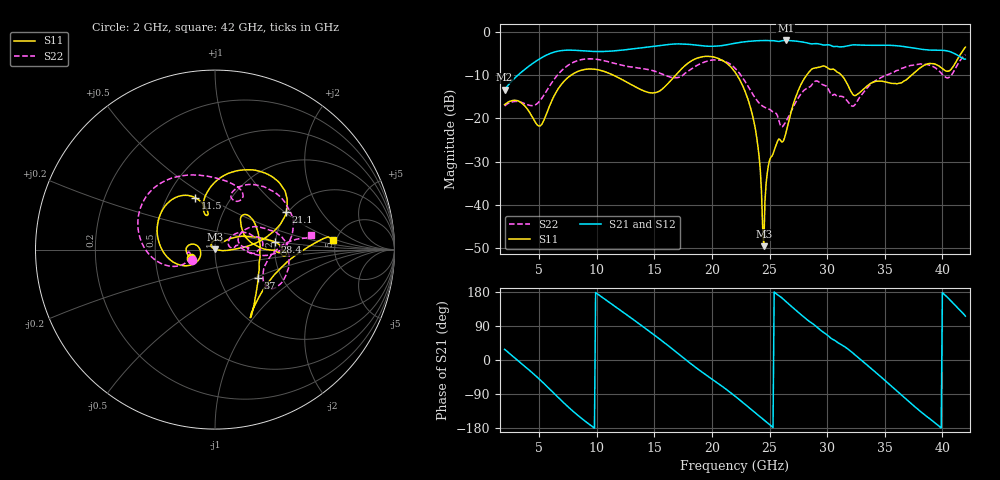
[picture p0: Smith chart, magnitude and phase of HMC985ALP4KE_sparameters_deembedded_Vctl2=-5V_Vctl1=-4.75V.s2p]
!s2p File: Measurements: S11, S21, S12, S22
# GHz S dB R 50.0
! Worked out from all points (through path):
!   401 points, 2 GHz to 42 GHz, reference 50 ohm
!   highest |S21| = -2.06 dB at 26.4 GHz (marker M1); lowest = -13.4 dB at 2 GHz (marker M2)
!   lowest |S11| = -49.5 dB at 24.5 GHz (marker M3), VSWR 1.01, Z = 49.8 + j0.275 ohm
!   |S11| at or under -10 dB: start of sweep to 7.808 GHz; 22.15 GHz to 28.24 GHz (6.082 GHz wide, 24.1 % of centre); 31.21 GHz to 37.36 GHz (6.148 GHz wide, 17.9 % of centre)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
!   |S22| runs from -22.0 to -5.4 dB; largest |S21 - S12| = 0.00096
!   S11 on the Smith chart (normalised r, x): 2 GHz: 0.76, -0.07; 11.5 GHz: 0.68, +0.44; 21.1 GHz: 1.96, +1.02; 28.4 GHz: 1.99, +0.19; 37 GHz: 1.52, -0.52; 42 GHz: 4.72, +0.86
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2  -16.88 -161.7  -13.43 28.3  -13.44 28.3  -17.18 -155.6
5  -21.80 -172.4  -6.37 -50.1  -6.38 -50.1  -16.18 -159.7
6.3  -14.84 -150.3  -4.76 -88.3  -4.76 -88.3  -11.03 -161.5
8.7  -8.91 150.4  -4.44 -154.5  -4.44 -154.5  -6.47 151.4
11.5  -10.16 111.1  -4.47 143.2  -4.47 143.2  -7.32 105.2
13.6  -13.11 101.2  -3.86 97.3  -3.86 97.3  -8.41 75.8
15.4  -13.81 105.8  -3.26 56.6  -3.26 56.6  -9.51 62.2
17.9  -7.34 80.3  -2.95 -3.4  -2.95 -3.3  -9.20 72.2
21.1  -6.97 27.7  -3.15 -74.2  -3.15 -74.2  -6.87 16.2
22  -9.36 17.1  -2.71 -95.4  -2.71 -95.4  -8.46 0.8
23.6  -20.27 0.0  -2.18 -135.1  -2.18 -135.0  -14.72 -4.2
24.5  -49.51 124.4  -2.08 -157.7  -2.08 -157.7  -17.38 8.2
25  -29.70 133.4  -2.11 -170.4  -2.11 -170.4  -17.95 10.9
26.4  -23.60 42.1  -2.06 154.9  -2.06 154.9  -20.85 33.2
28.4  -9.44 7.2  -2.72 102.9  -2.72 103.0  -12.88 18.7
28.7  -8.61 2.3  -2.86 96.7  -2.86 96.8  -12.19 16.7
30.7  -8.96 -2.8  -3.45 50.9  -3.45 50.9  -14.54 2.6
32.5  -14.70 32.0  -3.09 11.2  -3.09 11.2  -16.57 27.9
35.4  -11.82 19.3  -3.17 -64.3  -3.17 -64.3  -9.82 19.6
37  -10.84 -33.2  -3.60 -107.4  -3.60 -107.4  -8.03 5.3
39.8  -8.13 -57.0  -4.32 -176.8  -4.31 -176.8  -9.31 -35.2
42  -3.61 4.5  -6.36 115.6  -6.36 115.6  -5.35 8.9
